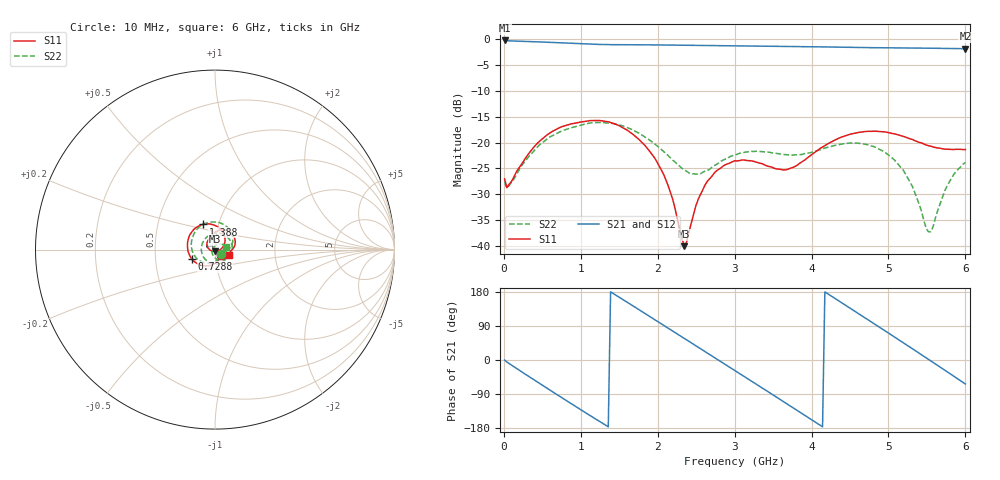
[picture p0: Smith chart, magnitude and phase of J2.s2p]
!Agilent Technologies,E8364B,MY43040528,A.07.50.67
!Agilent E8364B: A.07.50.67
!Date: Sunday, September 28, 2025 21:30:37
!Correction: S11(Full 2 Port(1,2))
!S21(Full 2 Port(1,2))
!S12(Full 2 Port(1,2))
!S22(Full 2 Port(1,2))
!S2P File: Measurements: S11, S21, S12, S22:
# Hz S  dB  R 50
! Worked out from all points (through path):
!   201 points, 10 MHz to 6 GHz, reference 50 ohm
!   highest |S21| = -0.36 dB at 10 MHz (marker M1); lowest = -1.9 dB at 6 GHz (marker M2)
!   group delay of S21, straight-line fit = 361 ps
!   lowest |S11| = -40.0 dB at 2.346 GHz (marker M3), VSWR 1.02, Z = 50.2 - j0.995 ohm
!   |S11| at or under -10 dB: start of sweep to end of sweep
!   |S22| runs from -37.2 to -16.1 dB; largest |S21 - S12| = 0.0026
!   S11 on the Smith chart (normalised r, x): 10 MHz: 1.07, -0.06; 728.8 MHz: 0.77, -0.08; 1.388 GHz: 0.84, +0.24; 6 GHz: 1.17, -0.07
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1e7  -27.02 -38.6  -0.36 -0.0  -0.38 0.1  -27.66 -39.6
3.995e7  -28.70 -22.2  -0.40 -5.4  -0.40 -5.3  -28.78 -23.8
3.9935e8  -20.73 -106.2  -0.61 -53.3  -0.60 -53.2  -21.47 -116.0
7.288e8  -17.11 -158.2  -0.80 -96.3  -0.79 -96.2  -17.94 -176.2
1.0283e9  -16.00 163.1  -1.02 -134.9  -1.01 -134.8  -16.55 137.7
1.3877e9  -16.14 115.8  -1.16 179.9  -1.15 179.9  -16.30 85.4
1.6872e9  -18.54 75.4  -1.18 141.7  -1.18 141.8  -17.66 46.0
2.01665e9  -24.45 30.2  -1.22 99.4  -1.22 99.4  -20.92 10.5
2.3461e9  -39.96 -80.7  -1.28 57.0  -1.28 57.0  -25.29 -5.8
2.61565e9  -28.17 167.7  -1.33 22.2  -1.33 22.3  -25.51 -1.4
3.005e9  -23.52 121.7  -1.40 -28.0  -1.39 -27.9  -22.41 -32.8
3.27455e9  -23.77 100.0  -1.43 -62.9  -1.43 -62.8  -21.69 -71.9
3.51415e9  -24.96 92.9  -1.46 -94.0  -1.46 -94.0  -22.04 -115.1
3.75375e9  -24.83 99.2  -1.50 -125.3  -1.50 -125.3  -22.43 -166.4
4.0233e9  -22.10 98.2  -1.56 -160.6  -1.55 -160.5  -21.77 132.0
4.29285e9  -19.61 82.9  -1.63 164.1  -1.63 164.2  -20.59 76.8
4.59235e9  -18.11 59.9  -1.71 124.8  -1.71 124.9  -20.13 22.9
5.01165e9  -18.14 26.3  -1.78 69.6  -1.77 69.7  -22.53 -47.0
5.31115e9  -19.42 7.0  -1.81 29.7  -1.81 29.8  -28.46 -103.5
5.5208e9  -20.62 -1.2  -1.85 1.6  -1.84 1.7  -37.21 164.5
5.7604e9  -21.29 -7.6  -1.89 -30.8  -1.88 -30.7  -28.43 54.6
6e9  -21.35 -19.5  -1.94 -63.4  -1.94 -63.3  -23.83 13.8
